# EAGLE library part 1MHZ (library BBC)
1MHz Bus
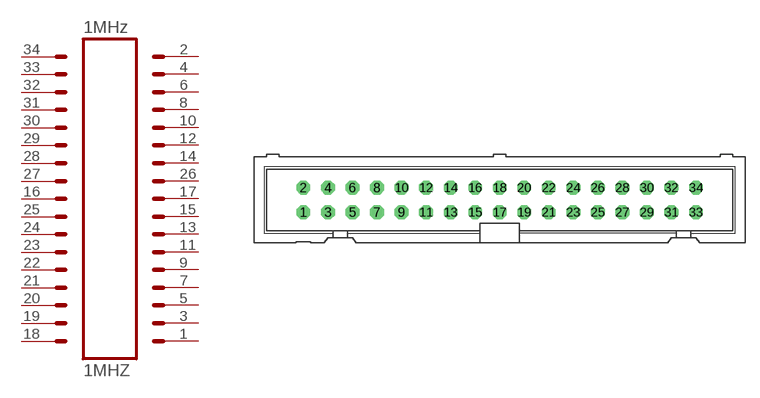
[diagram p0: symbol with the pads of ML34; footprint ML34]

Designator prefix -

## 1MHZ  [ML34]
1  1_GND  pas
2  2_RW  pas
3  3_GND  pas
4  4_1MHZ  pas
5  5_GND  pas
6  6_NMI  pas
7  7_GND  pas
8  8_IRQ  pas
9  9_GND  pas
10  10_FC  pas
11  11_GND  pas
12  12_FD  pas
13  13_GND  pas
14  14_RST  pas
15  15_GND  pas
16  16_ANALOG  pas
17  17_GND  pas
18  18_D0  pas
19  19_D1  pas
20  20_D2  pas
21  21_D3  pas
22  22_D4  pas
23  23_D5  pas
24  24_D6  pas
25  25_D7  pas
26  26_GND  pas
27  27_A0  pas
28  28_A1  pas
29  29_A2  pas
30  30_A3  pas
31  31_A4  pas
32  32_A5  pas
33  33_A6  pas
34  34_A7  pas

## Footprint ML34 (pad centres in mm)
HARTING
drill 0.914 octagon: 1 -20.32,-1.27; 2 -20.32,1.27; 3 -17.78,-1.27; 4 -17.78,1.27; 5 -15.24,-1.27; 6 -15.24,1.27; 7 -12.7,-1.27; 8 -12.7,1.27; 9 -10.16,-1.27; 10 -10.16,1.27; 11 -7.62,-1.27; 12 -7.62,1.27; 13 -5.08,-1.27; 14 -5.08,1.27; 15 -2.54,-1.27; 16 -2.54,1.27; 17 0,-1.27; 18 0,1.27; 19 2.54,-1.27; 20 2.54,1.27; 21 5.08,-1.27; 22 5.08,1.27; 23 7.62,-1.27; 24 7.62,1.27; 25 10.16,-1.27; 26 10.16,1.27; 27 12.7,-1.27; 28 12.7,1.27; 29 15.24,-1.27; 30 15.24,1.27; 31 17.78,-1.27; 32 17.78,1.27; 33 20.32,-1.27; 34 20.32,1.27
